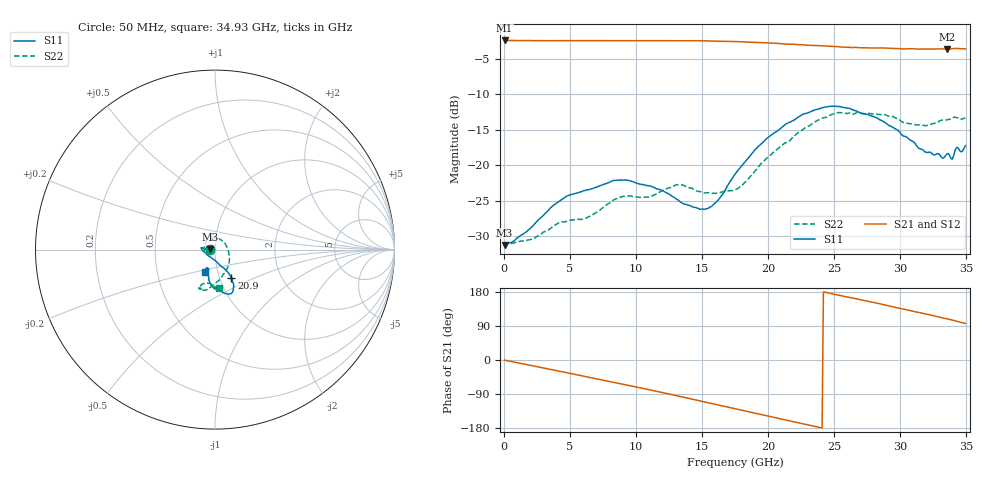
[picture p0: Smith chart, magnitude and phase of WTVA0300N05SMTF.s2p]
! 50 ohm 2-Port S-parameters measured by Modelithics Inc support@modelithics.com  Tampa, FL USA 813-866-6335 (February 2024)
! Smiths Interconnect,  3dB P/N: WTVA0300N05SMTF, Temperature: 75 C
! Board: 10 mil Rogers 4350B, Mounting Pad Dimensions: Length: 15 mils, Width: 25 mils, Gap: 40 mils.
# Hz S RI R 50
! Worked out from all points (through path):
!   352 points, 50 MHz to 34.93 GHz, reference 50 ohm
!   highest |S21| = -2.37 dB at 50 MHz (marker M1); lowest = -3.6 dB at 33.53 GHz (marker M2)
!   group delay of S21, straight-line fit = 21 ps
!   lowest |S11| = -31.2 dB at 50 MHz (marker M3), VSWR 1.06, Z = 47.3 + j0.0712 ohm
!   |S11| at or under -10 dB: start of sweep to end of sweep
!   |S22| runs from -31.4 to -12.5 dB; largest |S21 - S12| = 0.0089
!   S11 on the Smith chart (normalised r, x): 50 MHz: 0.95, +0.00; 20.9 GHz: 1.14, -0.37; 34.93 GHz: 0.87, -0.22
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5e7  -0.0274 0.000751  0.7613 -0.00412  0.7602 -0.0042  -0.0268 -0.000489
2.986e9  -0.0441 0.00342  0.7084 -0.2713  0.7073 -0.2719  -0.0321 -0.0104
4.6775e9  -0.0599 0.00472  0.6367 -0.4125  0.6357 -0.4119  -0.0353 -0.0189
5.8715e9  -0.0646 0.00878  0.5689 -0.502  0.5681 -0.5016  -0.0367 -0.0193
8.6575e9  -0.0779 0.0108  0.3633 -0.6657  0.3617 -0.6655  -0.0579 -0.00994
1.1742e10  -0.0673 -0.00695  0.0789 -0.7546  0.077 -0.7538  -0.0512 0.039
1.3135e10  -0.0545 -0.0174  -0.0596 -0.7566  -0.0617 -0.7555  -0.0381 0.0621
1.52245e10  -0.0237 -0.0429  -0.2674 -0.7077  -0.27 -0.7057  0.0175 0.0614
1.62195e10  -0.00453 -0.0566  -0.3591 -0.6609  -0.3597 -0.6595  0.0423 0.0476
1.7513e10  0.024 -0.0837  -0.4665 -0.5848  -0.4667 -0.5833  0.0655 0.0147
1.90055e10  0.0591 -0.1145  -0.5674 -0.4713  -0.5672 -0.4701  0.0806 -0.0431
2.0896e10  0.0917 -0.1557  -0.6581 -0.3018  -0.6574 -0.3008  0.0605 -0.1204
2.33835e10  0.1026 -0.2209  -0.6995 -0.0733  -0.6986 -0.073  -0.0103 -0.1979
2.61695e10  0.058 -0.2452  -0.6569 0.1775  -0.6555 0.1793  -0.0794 -0.2195
2.91545e10  -0.0251 -0.1889  -0.5332 0.4078  -0.5282 0.4124  -0.0821 -0.2063
3.1841e10  -0.0367 -0.1191  -0.3518 0.5616  -0.3481 0.5624  -0.0327 -0.1881
3.3234e10  -0.0415 -0.1039  -0.2364 0.6205  -0.232 0.6211  -0.00168 -0.2092
3.35325e10  -0.042 -0.113  -0.2112 0.6255  -0.2056 0.6264  0.00149 -0.2095
3.39305e10  -0.0422 -0.102  -0.1772 0.6416  -0.1717 0.6421  0.0118 -0.2138
3.4229e10  -0.0541 -0.1206  -0.1476 0.6529  -0.1415 0.6531  0.00957 -0.2171
3.4627e10  -0.0469 -0.1154  -0.1022 0.6581  -0.1015 0.6568  0.0137 -0.2114
3.49255e10  -0.0557 -0.1257  -0.0735 0.6596  -0.0724 0.6583  0.0228 -0.2144
